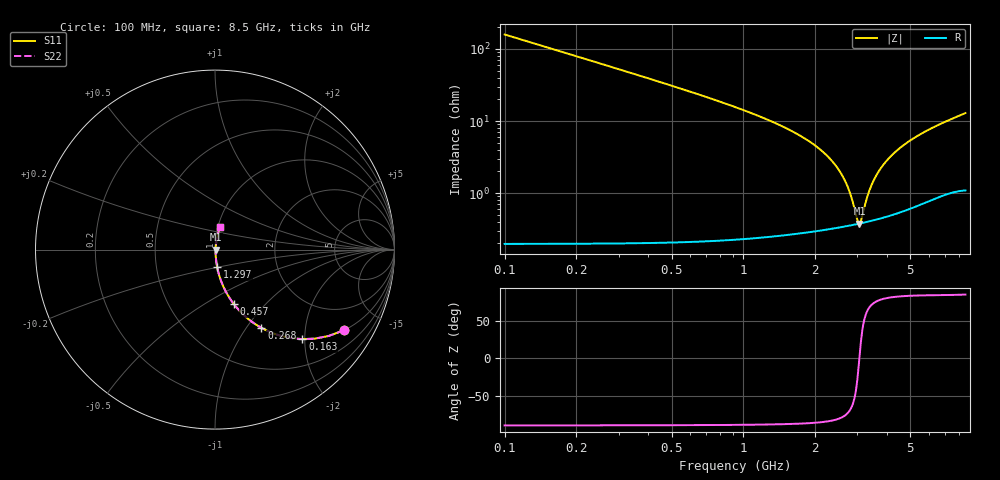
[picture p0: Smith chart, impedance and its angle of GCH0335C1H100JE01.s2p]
!Murata Part Number: GCH0335C1H100JE01
!These Parameters are Measured in Series Mode Connection
!Data Generated on Mar 13, 2026
!  o--ll--o
!Port1  Port2
!  o------o
!Operation Temp=25[degC], DC Bias Voltage=0[V]
!Freq. Start=100[MHz] Stop=9[GHz] 401[Steps]
# Hz S RI R 50
!Freq.(Hz) S11(Real) S11(Imag) S21(Real) S21(Imag) S12(Real) S12(Imag) S22(Real) S22(Imag)
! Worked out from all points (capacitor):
!   401 points, 100 MHz to 8.5 GHz, reference 50 ohm
!   read as one part in series: C = 10 pF near 142 MHz
!   lowest |Z| = 378 mohm at 3.061 GHz (marker M1)
!   series resonance near 3.058 GHz, so ESL is about 270 pH
!   S11 on the Smith chart (normalised r, x): 100 MHz: 1.00, -3.18; 163 MHz: 1.00, -1.95; 268 MHz: 1.00, -1.18; 457 MHz: 1.00, -0.68; 1.297 GHz: 1.00, -0.20; 8.5 GHz: 1.02, +0.26
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1e8  0.7163 -0.4502  0.2837 0.4502  0.2837 0.4502  0.7163 -0.4502
1.63e8  0.4866 -0.4988  0.5134 0.4988  0.5134 0.4988  0.4866 -0.4988
2.68e8  0.2584 -0.4361  0.7416 0.4361  0.7416 0.4361  0.2584 -0.4361
4.57e8  0.1053 -0.3039  0.8947 0.3039  0.8947 0.3039  0.1053 -0.3039
7.93e8  0.0358 -0.1799  0.9642 0.1799  0.9642 0.1799  0.0358 -0.1799
1.297e9  0.0124 -0.099  0.9876 0.099  0.9876 0.099  0.0124 -0.099
1.507e9  0.00889 -0.0789  0.9911 0.0789  0.9911 0.0789  0.00889 -0.0789
2.074e9  0.00469 -0.041  0.9953 0.041  0.9953 0.041  0.00469 -0.041
2.452e9  0.0038 -0.023  0.9962 0.023  0.9962 0.023  0.0038 -0.023
2.725e9  0.00363 -0.0119  0.9964 0.0119  0.9964 0.0119  0.00363 -0.0119
2.914e9  0.00366 -0.00499  0.9963 0.00499  0.9963 0.00499  0.00366 -0.00499
2.998e9  0.00371 -0.00205  0.9963 0.00205  0.9963 0.00205  0.00371 -0.00205
3.061e9  0.00376 9.73e-05  0.9962 -9.73e-05  0.9962 -9.73e-05  0.00376 9.73e-05
3.124e9  0.00382 0.0022  0.9962 -0.0022  0.9962 -0.0022  0.00382 0.0022
3.334e9  0.00409 0.00893  0.9959 -0.00893  0.9959 -0.00893  0.00409 0.00893
3.544e9  0.00445 0.0153  0.9956 -0.0153  0.9956 -0.0153  0.00445 0.0153
3.859e9  0.00514 0.0242  0.9949 -0.0242  0.9949 -0.0242  0.00514 0.0242
4.3e9  0.00636 0.0359  0.9936 -0.0359  0.9936 -0.0359  0.00636 0.0359
4.909e9  0.00849 0.0507  0.9915 -0.0507  0.9915 -0.0507  0.00849 0.0507
5.707e9  0.0119 0.0684  0.9881 -0.0684  0.9881 -0.0684  0.0119 0.0684
7.114e9  0.0191 0.0969  0.9809 -0.0969  0.9809 -0.0969  0.0191 0.0969
8.5e9  0.0265 0.1237  0.9735 -0.1237  0.9735 -0.1237  0.0265 0.1237
